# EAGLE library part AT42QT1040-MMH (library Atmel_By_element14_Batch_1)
QTouch 4-Key Sensor IC
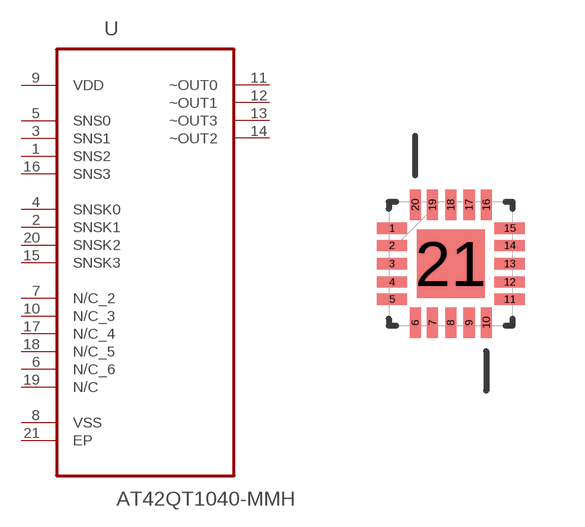
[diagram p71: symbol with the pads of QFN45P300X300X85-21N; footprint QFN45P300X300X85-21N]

Designator prefix U

## AT42QT1040-MMH (MPN: AT42QT1040-MMH; OC_FARNELL: 1748487; OC_NEWARK: 26R5669; PACKAGE: QFN-20; SUPPLIER: Atmel)  [QFN45P300X300X85-21N]
1  SNS2
2  SNSK1
3  SNS1
4  SNSK0
5  SNS0
6  N/C_6
7  N/C_2  nc
8  VSS  pas
9  VDD  pwr
10  N/C_3  nc
11  ~OUT0  out
12  ~OUT1  out
13  ~OUT3  out
14  ~OUT2  out
15  SNSK3  out
16  SNS3
17  N/C_4  nc
18  N/C_5  nc
19  N/C  nc
20  SNSK2
21  EP  pas

## Footprint QFN45P300X300X85-21N (pad centres in mm)
smd 0.762 x 0.279: 1 -1.473,0.889; 2 -1.473,0.457; 3 -1.473,0; 4 -1.473,-0.457; 5 -1.473,-0.889; 11 1.473,-0.889; 12 1.473,-0.457; 13 1.473,0; 14 1.473,0.457; 15 1.473,0.889
smd 0.279 x 0.762: 6 -0.889,-1.473; 7 -0.457,-1.473; 8 0,-1.473; 9 0.457,-1.473; 10 0.889,-1.473; 16 0.889,1.473; 17 0.457,1.473; 18 0,1.473; 19 -0.457,1.473; 20 -0.889,1.473
smd 1.702 x 1.702: 21 0,0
